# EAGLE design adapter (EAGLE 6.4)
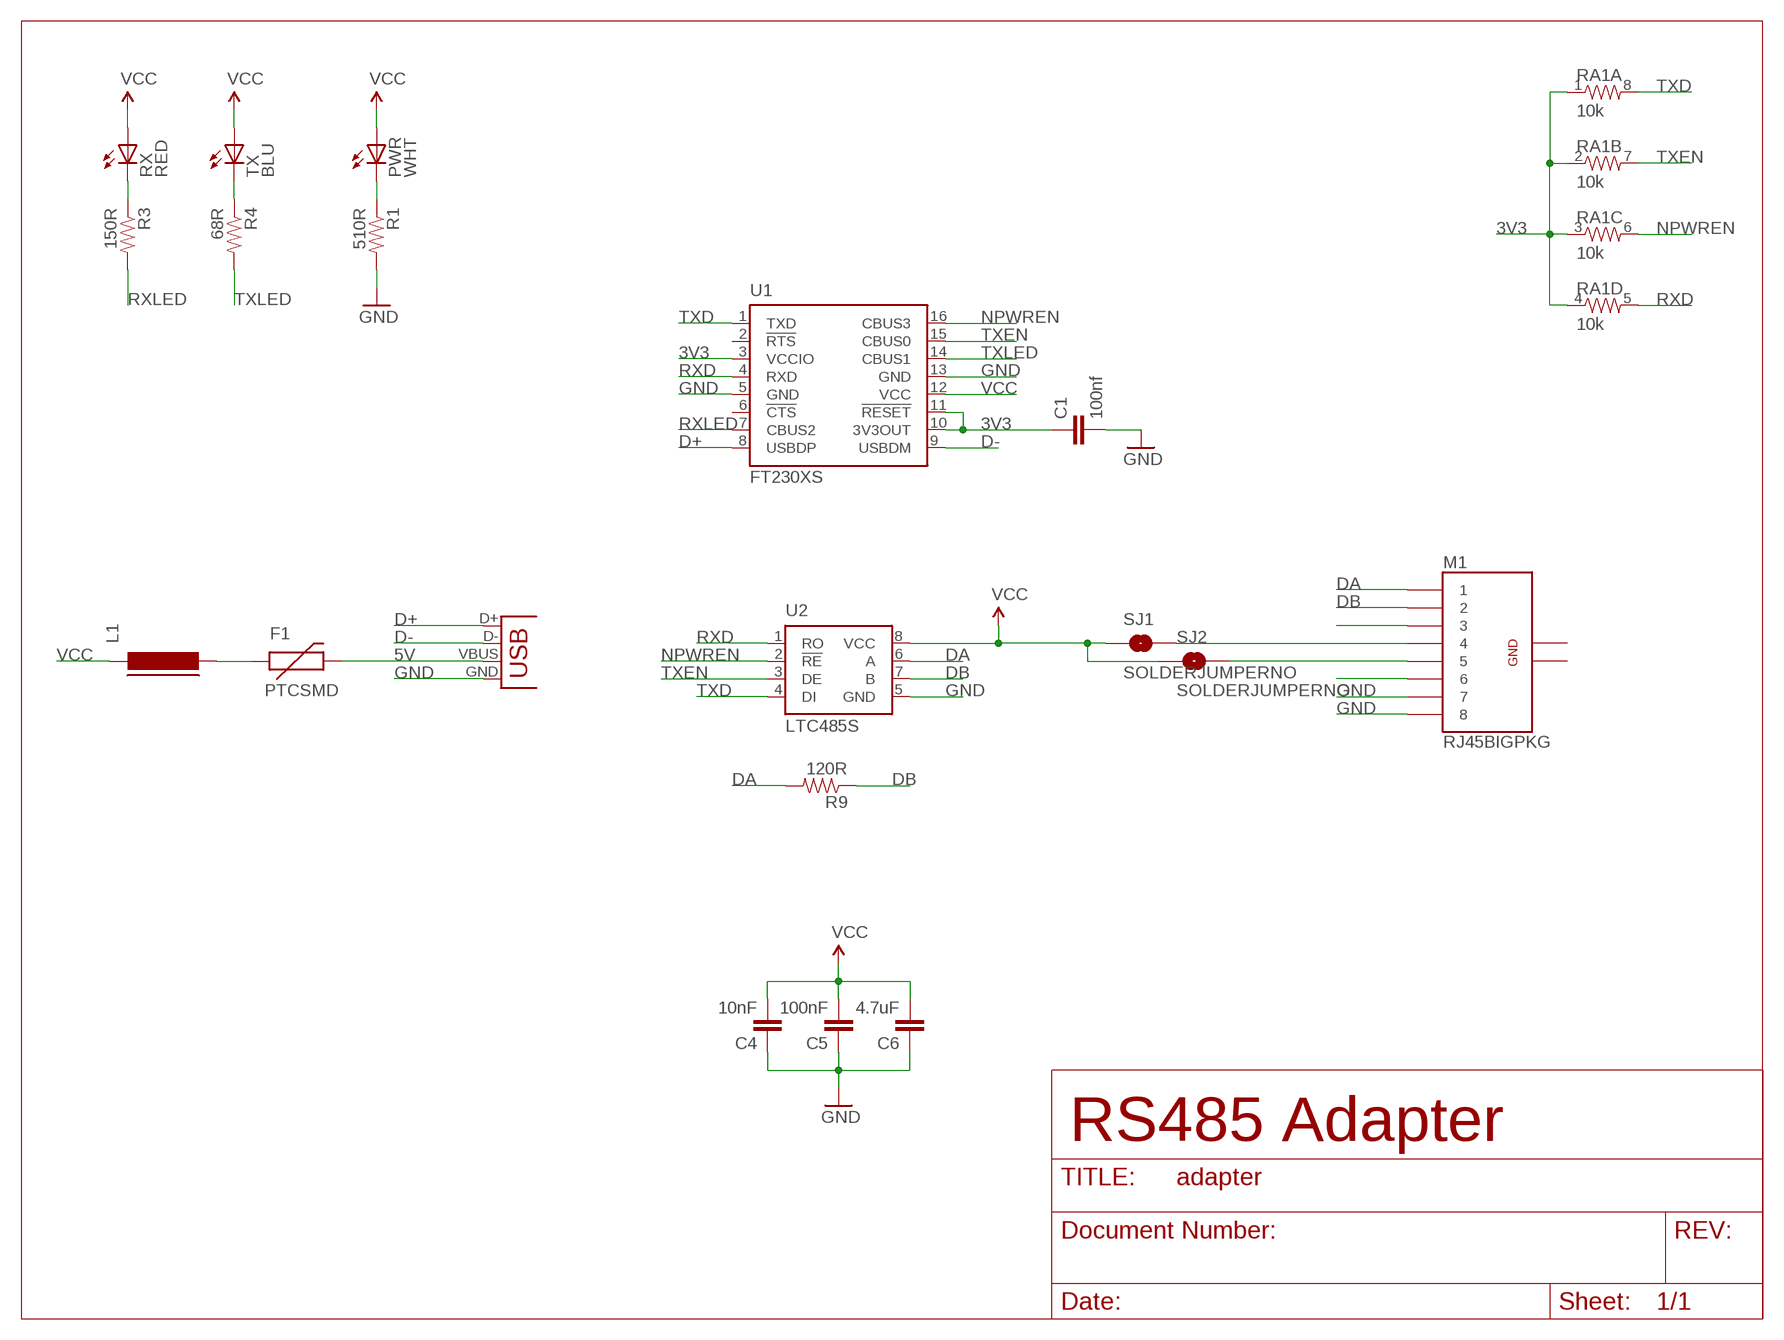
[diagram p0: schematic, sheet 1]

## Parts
C1  100nf  CAP0603-CAP  [0603-CAP]
C4  10nF  CAP0603-CAP  [0603-CAP]
C5  100nF  CAP0603-CAP  [0603-CAP]
C6  4.7uF  CAP0603-CAP  [0603-CAP]
F1  PTCSMD  [PTC-1206]
L1  FERRITE-0603  [FB603]
M1  RJ45BIGPKG  [RJ45-8_SMD-1]
M2  USBSMD  [USB-MINIB]
PWR  WHT  LED0603  [LED-0603]
R1  510R  RESISTOR0603-RES  [0603-RES]
R3  150R  RESISTOR0603-RES  [0603-RES]
R4  68R  RESISTOR0603-RES  [0603-RES]
R9  120R  RESISTOR0603-RES  [0603-RES]
RA1  10k  RES-ARRAY  [0603-ARV-4]
RX  RED  LED0603  [LED-0603]
SJ1  SOLDERJUMPERNO  [SJ_2S-NO]
SJ2  SOLDERJUMPERNO  [SJ_2S-NO]
TX  BLU  LED0603  [LED-0603]
U1  FT230XS  [SSOP16]
U2  LTC485S  [SOIC8]

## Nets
3V3: C1.1 RA1.1 RA1.2 RA1.3 RA1.4 U1.3(VCCIO) U1.10(3V3OUT) U1.11(!RESET)
5V: F1.2 M2.VBUS
D+: M2.D+ U1.8(USBDP)
D-: M2.D- U1.9(USBDM)
DA: M1.P$1 R9.2 U2.6(A)
DB: M1.P$2 R9.1 U2.7(B)
GND: C1.2 C4.1 C5.1 C6.1 M1.P$7 M1.P$8 M2.GND R1.2 U1.5(GND) U1.13(GND) U2.5(GND)
N$1: M1.P$6
N$2: M1.P$3
N$3: R3.1 RX.C
N$4: R4.1 TX.C
N$5: F1.1 L1.2
N$6: PWR.C R1.1
N$11: M1.P$5 SJ2.2
N$12: M1.P$4 SJ1.2
NPWREN: RA1.6 U1.16(CBUS3) U2.2(!RE)
RXD: RA1.5 U1.4(RXD) U2.1(RO)
RXLED: R3.2 U1.7(CBUS2)
TXD: RA1.8 U1.1(TXD) U2.4(DI)
TXEN: RA1.7 U1.15(CBUS0) U2.3(DE)
TXLED: R4.2 U1.14(CBUS1)
VCC: C4.2 C5.2 C6.2 L1.1 PWR.A RX.A SJ1.1 SJ2.1 TX.A U1.12(VCC) U2.8(VCC)
Unconnected: M1.P$9(GND0) M1.P$10(GND1) U1.2(!RTS) U1.6(!CTS)

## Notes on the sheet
- RS485 Adapter

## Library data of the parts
C1 C4-C6 = SparkFun:CAP: Capacitor
F1 = SparkFun:PTC: Resettable Fuse PTC
L1 = dp_devices:FERRITE: Ferrite bead in various packages
M1 = Protofusion:RJ45: RJ45 Jack Simple RJ45, 8-pin connection - connector for common Cat5, Cat5e, and Cat6 Ethernet cables. MOLEX SMD P/N: 43743-8101
M2 = SparkFun:USB: USB Connectors USB-B-PTH is fully proven SKU : PRT-00139 USB-miniB is fully proven SKU : PRT-00587 USB-A-PCB is untested. USB-A-H is throughly reviewed, but untested. Spark Fun Electronics SKU : PRT-00437 USB-B-SMT is throughly reviewed, but untested. Needs silkscreen touching up. USB-A-S has not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
PWR RX TX = SparkFun:LED: LEDs
R1 R3 R4 R9 = SparkFun:RESISTOR: Resistor
RA1 = Protofusion:RES-ARRAY
SJ1 SJ2 = SparkFun:SOLDERJUMPER: Solder Jumper
U1 = ftdichip:FT230X: USB to BASIC UART IC Auto generated by make-symbol-device-package-bsdl.ulp Rev. 43 Source: Data sheet
U2 = linear-technology:LTC485: Low Power RS485 Interface Transceiver Source: http://www.linear.com/pc/downloadDocument.do?navId=H0,C1,C1007,C1017,P2064,D1718; OC_FARNELL: unknown; OC_NEWARK: unknown

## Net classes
0 default: width 0.254 mm
1 power: width 0.508 mm

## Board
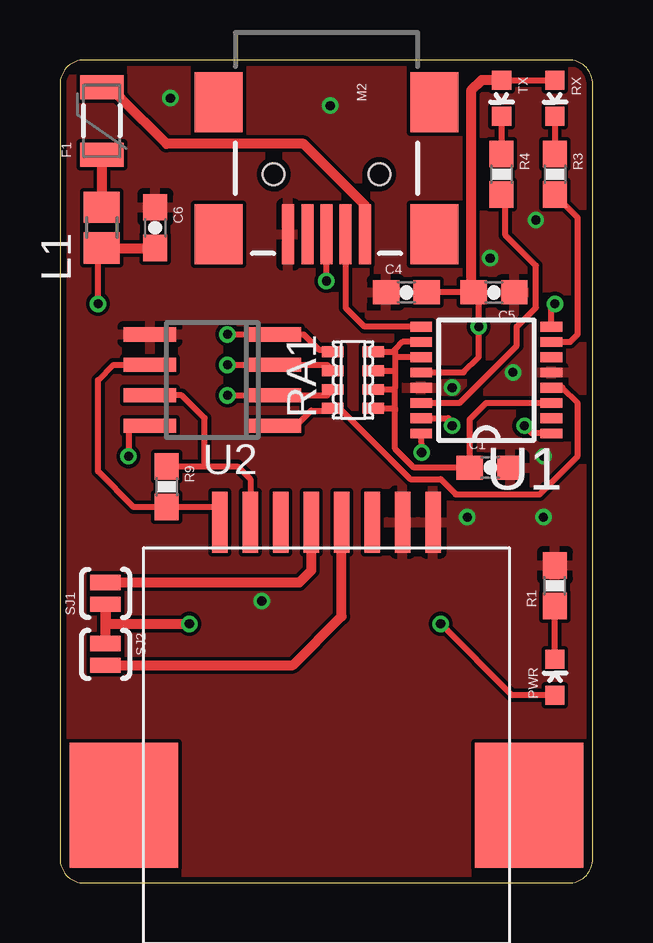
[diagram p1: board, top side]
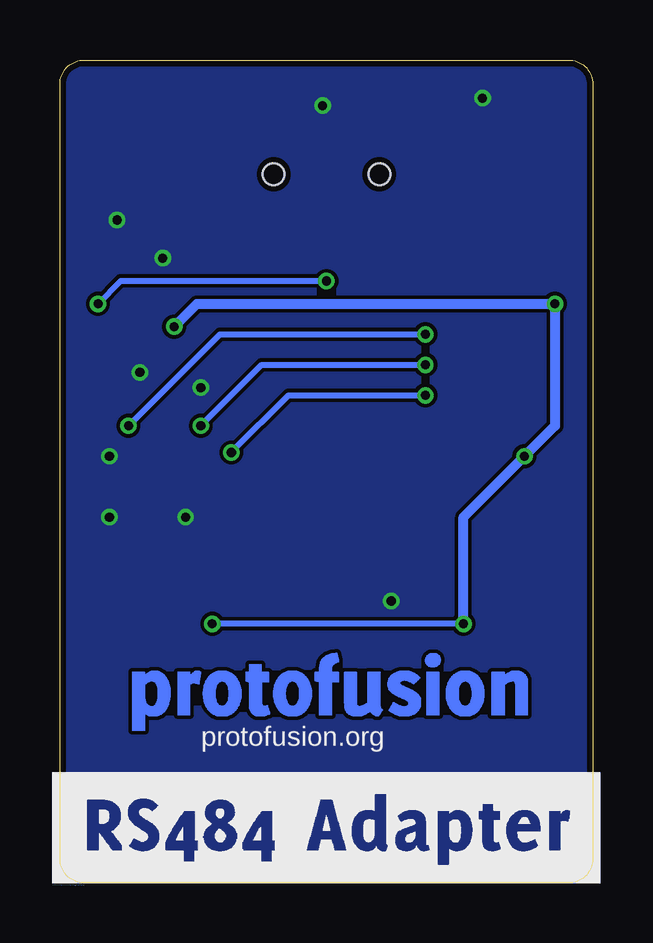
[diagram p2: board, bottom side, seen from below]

Size 22.23 x 34.29 mm. Coordinates in mm from the lower left corner, seen from the top.
Outline: 0,33.27 0,1.02 arc90 1.02,0 21.21,0 arc90 22.23,1.02 22.23,33.27 arc90 21.21,34.29 1.02,34.29 arc90 0,33.27
Copper layers (1*16): Top 0.035mm / dielectric 1.5mm / Bottom 0.035mm
Design rules "ITead_rule": minimum track width 6mil, minimum drill 12mil, track to track 6mil, track to pad 6mil, pad to pad 6mil, via to via 6mil, smd to smd 0mil, copper to edge 10mil, drill to drill 10mil, minimum pad ring 10mil, minimum via ring 6mil, stop-mask expansion 2mil, vias tented up to drill 100mil, thermal gap 10mil

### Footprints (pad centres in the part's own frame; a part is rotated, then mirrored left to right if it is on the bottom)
0603-CAP = smd 1.1 x 1: 1 -0.85,0; 2 0.85,0
PTC-1206 = smd 1 x 1.8: 1 -1.4,0; 2 1.4,0
FB603 = smd 1.3 x 1.5: 1 -0.85,0; 2 0.85,0
RJ45-8_SMD-1 = smd 0.635 x 2.54: P$1 -4.445,9.957; P$2 -3.175,9.957; P$3 -1.905,9.957; P$4 -0.635,9.957; P$5 0.635,9.957; P$6 1.905,9.957; P$7 3.175,9.957; P$8 4.445,9.957 | smd 4.521 x 5.207: P$9 8.445,-1.841; P$10 -8.445,-1.841
USB-MINIB = smd 2.5 x 0.5: D+ 2.5,0; D- 2.5,0.8; GND 2.5,-1.6; ID 2.5,-0.8; VBUS 2.5,1.6 | smd 2.5 x 2: MTN1 -3,4.5; MTN2 2.5,4.5; MTN3 -3,-4.5; MTN4 2.5,-4.5 | hole 0.9: 0,2.2; 0,-2.2
LED-0603 = smd 0.8 x 0.8: A 0,-0.75; C 0,0.75
0603-RES = smd 1.1 x 1: 1 -0.85,0; 2 0.85,0
0603-ARV-4 = smd 0.457 x 0.902: 1 -1.181,0.845; 2 -0.394,0.845; 3 0.394,0.845; 4 1.181,0.845; 5 1.181,-0.845; 6 0.394,-0.845; 7 -0.394,-0.845; 8 -1.181,-0.845
SJ_2S-NO = smd 0.635 x 1.27: 1 -0.45,0; 2 0.45,0
SSOP16 = smd 0.914 x 0.406: 1 -2.718,2.223; 2 -2.718,1.587; 3 -2.718,0.953; 4 -2.718,0.318; 5 -2.718,-0.318; 6 -2.718,-0.953; 7 -2.718,-1.587; 8 -2.718,-2.223; 9 2.718,-2.223; 10 2.718,-1.587; 11 2.718,-0.953; 12 2.718,-0.318; 13 2.718,0.318; 14 2.718,0.953; 15 2.718,1.587; 16 2.718,2.223
SOIC8 = smd 0.6 x 2.2: 1 -1.905,-2.6; 2 -0.635,-2.6; 3 0.635,-2.6; 4 1.905,-2.6; 5 1.905,2.6; 6 0.635,2.6; 7 -0.635,2.6; 8 -1.905,2.6

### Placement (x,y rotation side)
C1  17.94,17.3 0 top
C4  14.45,24.61 0 top
C5  18.1,24.61 180 top
C6  3.97,27.3 270 top
F1  1.75,31.75 90 top
L1  1.75,27.3 90 top
M1  11.11,5.08 0 top
M2  11.11,29.53 270 top
PWR  20.64,8.57 0 top
R1  20.64,12.38 90 top
R3  20.64,29.53 270 top
R4  18.41,29.53 270 top
R9  4.45,16.51 270 top
RA1  12.22,20.95 270 top
RX  20.64,32.7 180 top
SJ1  1.91,12.07 90 top
SJ2  1.91,9.53 270 top
TX  18.41,32.7 180 top
U1  17.78,20.95 180 top
U2  6.35,20.95 90 top
U$3  [RS485-ADAPTER-LOGO-SILK]  22.54,0 0 bottom
U$4  [PROTOFUSION_LOGO_STOP]  19.21,6.35 0 bottom

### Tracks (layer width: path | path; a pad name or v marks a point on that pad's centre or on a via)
3V3
  Top 0.254: U1.10 14.29,22.54 13.97,22.22 | 13.97,22.22 13.97,21.91 | 13.97,21.91 13.97,21.27 | 13.97,21.27 13.97,20.64 | RA1.3 13.89,20.56 13.97,20.64 | RA1.2 13.89,21.35 13.97,21.27 | RA1.1 13.88,22.14 13.97,22.22 | U1.11 13.97,21.91 | 13.97,19.77 13.97,20.64 | U1.3 17.78,20 17.09,19.31 C1.1 14.76,17.3 13.97,18.1 13.97,19.68 13.97,19.77 | RA1.4 13.97,19.77
5V
  Top 0.406: M2.VBUS 12.71,28.24 10.16,30.8 4.45,30.8 2.54,32.7 1.88,33.34 F1.2
D+  (via drill 0.38)
  Top 0.254: U1.8 20.5,23.99 v20.64,24.13 | v11.11,25.08 M2.D+
  Bottom 0.254: v20.64,24.13 19.68,25.08 v11.11,25.08
D-
  Top 0.254: U1.9 12.7,23.18 11.91,23.97 M2.D-
DA
  Top 0.254: M1.P$1 6.67,15.66 R9.2 3.07,15.66 1.59,17.15 1.59,20.95 2.22,21.59 U2.6
DB
  Top 0.254: M1.P$2 7.94,16.83 7.41,17.36 R9.1 6.03,17.36 6.03,19.37 5.08,20.32 U2.7
GND  (via drill 0.38)
  other vias: 16.35,20.64 20.16,17.78 19.84,27.62 17.94,26.04 4.6,32.7 11.27,32.39 18.89,21.27 16.99,15.24 8.41,11.75 20.16,15.24
  pour Bottom: -35.88,53.02 66.04,54.29 63.18,-28.89 -38.73,-30.16
  pour Top: -34.61,54.29 61.28,53.98 59.05,-34.92 -36.83,-34.61
N$3
  Top 0.254: RX.C R3.1
N$4
  Top 0.254: TX.C R4.1
N$5
  Top 0.406: F1.1 L1.2
N$6
  Top 0.254: PWR.C R1.1
N$11
  Top 0.406: SJ2.2 9.71,9.08 11.75,11.11 M1.P$5
N$12
  Top 0.406: M1.P$4 10.48,13.02 9.97,12.51 SJ1.2
NPWREN  (via drill 0.38)
  Top 0.254: RA1.6 11.14,20.32 U2.2 v6.99,20.32 | U1.16 v15.08,17.94
  Bottom 0.254: v15.08,17.94 12.7,20.32 v6.99,20.32
RXD
  Top 0.254: U2.1 9.84,19.05 10.48,19.68 11.29,19.68 RA1.5 11.66,19.77 14.61,16.83 15.88,16.83 16.51,16.19 20,16.19 21.59,17.78 21.59,20 20.95,20.64 U1.4
RXLED
  Top 0.254: U1.7 21.27,22.54 21.59,22.86 21.59,27.72 R3.2
TXD  (via drill 0.38)
  Top 0.254: RA1.8 11.29,22.22 10.79,22.22 10.16,22.86 U2.4 v6.99,22.86 | U1.1 19.68,18.73 v19.37,19.05
  Bottom 0.254: v19.37,19.05 15.56,22.86 v6.99,22.86
TXEN  (via drill 0.38)
  Top 0.254: RA1.7 11.14,21.59 U2.3 v6.99,21.59 | U1.15 16.19,19.37 16.35,19.21 v16.35,19.05
  Bottom 0.254: v16.35,19.05 13.81,21.59 v6.99,21.59
TXLED
  Top 0.254: U1.14 16.67,20 19.05,22.38 19.05,23.18 19.84,23.97 19.84,25.72 18.57,26.99 18.57,28.52 R4.2
VCC  (via drill 0.38)
  Top 0.254: TX.A RX.A | U1.12 16.83,21.27 17.46,21.91 v17.46,23.18 17.46,24.39 C5.2 C4.2 | U2.8 2.86,19.05 v2.86,17.78 | v1.59,24.13 1.59,26.3 L1.1 | PWR.A 18.85,7.82 v15.88,10.79
  Top 0.406: L1.1 C6.2 | SJ2.1 SJ1.1 1.91,10.79 v5.4,10.79 | TX.A 17.58,33.45 17.14,33.02 17.14,24.71 C5.2
  Bottom 0.254: v5.4,10.79 v15.88,10.79
  Bottom 0.406: v5.4,10.79 5.4,15.24 v2.86,17.78 1.59,19.05 v1.59,24.13 16.51,24.13 v17.46,23.18

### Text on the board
bPlace: protofusion.org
